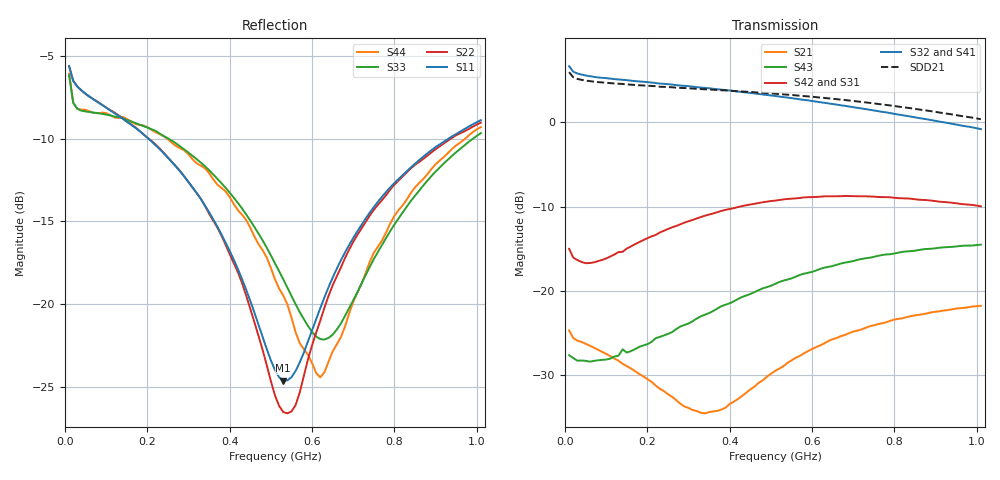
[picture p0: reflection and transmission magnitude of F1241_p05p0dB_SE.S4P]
! Integrated Device Technology
! Corporate Headquarters
! 6024 Silver Creek Valley Road
! San Jose, CA 95138  USA
! Phone:  1-408-284-8200
! Toll Free:  1-800-223-1366
! Webpage:  http://www.idt.com/
! Timing and RF Division
! 515 Groton Road, Suite 102
! Westford, MA 01886-6024
! Device:  F1241
! Description: Dual Intermediate Frequency Digital Variable Gain Amplifier
! Frequency:  10.0 -  500.00 MHz
! Package:  5x5 mm QFN Plastic Package: 32 pin
! Ports:  8 RF, 20 DC
!  Pin  1  = GA3  Pin 17  = RF OUT_B+
!  Pin  2  = GA4  Pin 18  = RF OUT_B-
!  Pin  3  = GA5  Pin 19  = STBY_B
!  Pin  4  = ISET_A  Pin 20  = Ground
!  Pin  5  = ISET_B  Pin 21  = Ground
!  Pin  6  = GB5  Pin 22  = STB_A
!  Pin  7  = GB4  Pin 23  = RF OUT_A-  = Port 4
!  Pin  8  = GB3  Pin 24  = RF OUT_A+  = Port 3
!  Pin  9  = GB2  Pin 25  = NO CONNECT
!  Pin 10  = GB1  Pin 26  = NO CONNECT
!  Pin 11  = RF IN_B+  Pin 27  = VCC
!  Pin 12  = RF IN_B-  Pin 28  = Ground
!  Pin 13  = Ground  Pin 29  = RF IN_A-  = Port 2
!  Pin 14  = VCC  Pin 30  = RF IN_A+  = Port 1
!  Pin 15  = NO CONNECT  Pin 31  = GA1
!  Pin 16  = NO CONNECT  Pin 32  = GA2
! State:  15
! Gain State:  5.0 dB
! Voltages:  Vcc = +5.00 Volts  Icc approximately 160.0 mA or 80 mA per channel.
! Data:  The device was measured on a custom evaluation board which has
!  individual transmission lines to the RF pins.  Data was collected
!  using a calibrated network analyzer.  The evaluation board was
!  de-embedded using a port reference technique.
!  The reference plane is the edge of the package pin.
!  Only Channel A was measured.
!  This data is in single-ended operation.  If your needs are balanced
!  or differential S-parameters then this file needs to be used a
!  linear simulator.
! Misc:  Lot Code  160028MY
!  Action Tracker AT004
! Date Measured:  2014-08-14
! Date:  2014-08-28  MJV
! Note:
!  Integrated Device Technology supplies this data as a sample of measured
!  data at the package pin for this product.  Your particular data for this
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# Hz S dB R 50
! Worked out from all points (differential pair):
!   101 points, 10 MHz to 1.01 GHz, reference 50 ohm
!   strongest paths, dB at 10 MHz, 260 MHz, 510 MHz, 760 MHz, 1.01 GHz:
!     S32: 6.6, 4.5, 3.1, 1.3, -0.8
!     S41: 6.7, 4.4, 3.0, 1.2, -1.0
!     S42: -15.0, -12.5, -9.3, -8.9, -10.0
!     S31: -15.0, -12.4, -9.3, -8.9, -10.1
!     S43: -27.6, -24.9, -19.2, -15.8, -14.5
!     S21: -24.7, -32.5, -29.5, -23.9, -21.8
!   taken as a pair (ports 2,1 in; 3,4 out), SDD21 dB: 5.9, 4.1, 3.4, 2.2, 0.4
!   lowest |S11| = -24.6 dB at 530 MHz (marker M1), VSWR 1.12, Z = 45.9 - j3.83 ohm
!   |S11| at or under -10 dB: 202.3 MHz to 931.7 MHz (729.4 MHz wide, 129 % of centre)
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1e7  -5.62 -18.2  -24.66 -20.7  -44.51 4.7  -18.18 13.8
     -24.67 -20.7  -5.63 -18.0  -18.20 13.4  -44.49 5.0
     -14.99 160.7  6.64 174.2  -6.16 -27.4  -27.72 -174.2
     6.67 174.3  -15.00 160.8  -27.61 -174.3  -6.09 -27.4
4e7  -7.09 -14.8  -26.03 -13.8  -44.25 21.8  -18.19 -1.2
     -26.04 -13.8  -7.09 -14.5  -18.18 -0.9  -44.12 20.5
     -16.54 145.5  5.64 169.8  -8.31 -11.6  -28.44 171.4
     5.66 169.7  -16.56 145.6  -28.24 171.2  -8.25 -11.1
3.3e8  -13.66 -51.1  -33.95 9.6  -33.04 41.0  -18.49 -20.6
       -34.44 6.6  -13.65 -47.4  -18.44 -20.2  -33.04 39.7
       -11.25 49.4  4.10 128.6  -11.46 -35.6  -23.43 122.2
       4.07 127.9  -11.23 49.2  -23.00 121.8  -11.64 -33.3
5.3e8  -24.65 -134.7  -28.42 46.2  -29.78 27.5  -18.29 -34.9
       -28.93 48.8  -26.54 -129.3  -18.12 -34.6  -29.77 25.1
       -9.20 9.3  2.98 102.2  -18.51 -74.2  -19.22 94.1
       2.90 101.2  -9.15 8.4  -18.78 93.1  -19.49 -70.3
6.2e8  -20.26 160.3  -26.13 44.8  -28.76 20.9  -18.35 -42.2
       -26.45 47.3  -21.01 155.3  -18.11 -41.9  -28.74 18.1
       -8.88 -6.4  2.37 90.9  -22.13 -123.9  -17.79 81.3
       2.27 89.9  -8.82 -7.6  -17.38 80.8  -24.44 -133.0
8e8  -12.69 128.2  -23.44 34.7  -27.16 7.1  -18.76 -57.0
     -23.39 37.1  -12.78 126.1  -18.41 -56.6  -27.22 3.9
     -9.04 -34.0  0.99 69.7  -15.20 156.8  -15.87 57.9
     0.85 68.8  -8.95 -36.1  -15.56 57.2  -14.67 149.3
1.01e9  -8.88 114.8  -21.90 22.5  -26.01 -9.5  -19.73 -71.9
        -21.76 24.2  -9.03 114.0  -19.18 -72.1  -26.02 -13.5
        -10.09 -59.1  -0.83 47.9  -9.67 134.4  -14.87 34.1
        -1.01 47.1  -9.97 -62.0  -14.51 33.5  -9.31 130.2
